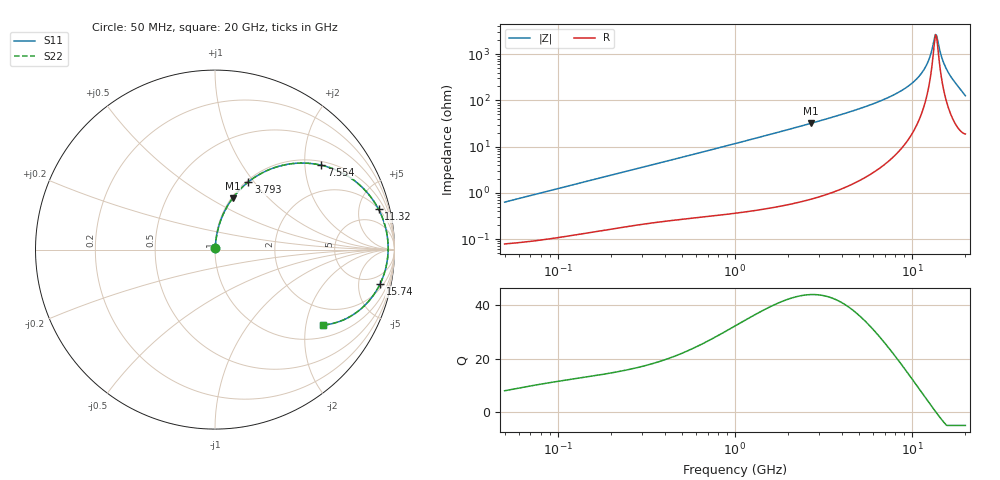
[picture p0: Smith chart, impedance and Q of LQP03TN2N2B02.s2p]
!Murata Part Number: LQP03TN2N2B02
!These Parameters are Measured in Series Mode Connection
!  o--[Z]--o
!Port1  Port2
!  o-------o
!Freq. Start=50[MHz] Stop=20[GHz], 401[Steps]
# Hz S RI R 50
!Freq.(Hz) S11(Real) S11(Imag) S21(Real) S21(Imag) S12(Real) S12(Imag) S22(Real) S22(Imag)
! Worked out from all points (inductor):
!   401 points, 50 MHz to 20 GHz, reference 50 ohm
!   read as one part in series: L = 1.98 nH near 51.52 MHz
!   highest Q = 43.9 at 2.687 GHz (marker M1), where L = 1.89 nH
!   self-resonance near 13.55 GHz
!   S11 on the Smith chart (normalised r, x): 50 MHz: 1.00, +0.01; 3.793 GHz: 1.02, +0.94; 7.554 GHz: 1.11, +2.43; 11.32 GHz: 2.04, +7.72; 15.74 GHz: 2.74, -8.90; 20 GHz: 1.37, -2.50
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5e7  0.000821 0.00623  0.9992 -0.00623  0.9992 -0.00623  0.000821 0.00623
1.364002e8  0.00157 0.0166  0.9984 -0.0166  0.9984 -0.0166  0.00157 0.0166
3.721004e8  0.00423 0.0435  0.9958 -0.0435  0.9958 -0.0435  0.00423 0.0435
1e9  0.0167 0.1136  0.9833 -0.1136  0.9833 -0.1136  0.0167 0.1136
2.687447e9  0.0979 0.286  0.9021 -0.286  0.9021 -0.286  0.0979 0.286
2.728004e9  0.1006 0.2897  0.8994 -0.2897  0.8994 -0.2897  0.1006 0.2897
3.792786e9  0.1853 0.3767  0.8147 -0.3767  0.8147 -0.3767  0.1853 0.3767
5.352748e9  0.3428 0.4603  0.6572 -0.4603  0.6572 -0.4603  0.3428 0.4603
7.442007e9  0.5804 0.4728  0.4196 -0.4728  0.4196 -0.4728  0.5804 0.4728
7.554318e9  0.5929 0.4701  0.4071 -0.4701  0.4071 -0.4701  0.5929 0.4701
9.600142e9  0.7969 0.3682  0.2031 -0.3682  0.2031 -0.3682  0.7969 0.3682
1.050288e10  0.8648 0.2972  0.1352 -0.2972  0.1352 -0.2972  0.8648 0.2972
1.131968e10  0.9116 0.2242  0.0884 -0.2242  0.0884 -0.2242  0.9116 0.2242
1.238412e10  0.9505 0.1218  0.0495 -0.1218  0.0495 -0.1218  0.9505 0.1218
1.334722e10  0.9643 0.0272  0.0357 -0.0272  0.0357 -0.0272  0.9643 0.0272
1.354865e10  0.9647 0.00764  0.0353 -0.00764  0.0353 -0.00764  0.9647 0.00764
1.375312e10  0.9643 -0.0121  0.0357 0.0121  0.0357 0.0121  0.9643 -0.0121
1.396067e10  0.9631 -0.032  0.0369 0.032  0.0369 0.032  0.9631 -0.032
1.482269e10  0.9491 -0.112  0.0509 0.112  0.0509 0.112  0.9491 -0.112
1.573793e10  0.9198 -0.191  0.0802 0.191  0.0802 0.191  0.9198 -0.191
1.747767e10  0.827 -0.3182  0.173 0.3182  0.173 0.3182  0.827 -0.3182
2e10  0.6 -0.4206  0.4 0.4206  0.4 0.4206  0.6 -0.4206
